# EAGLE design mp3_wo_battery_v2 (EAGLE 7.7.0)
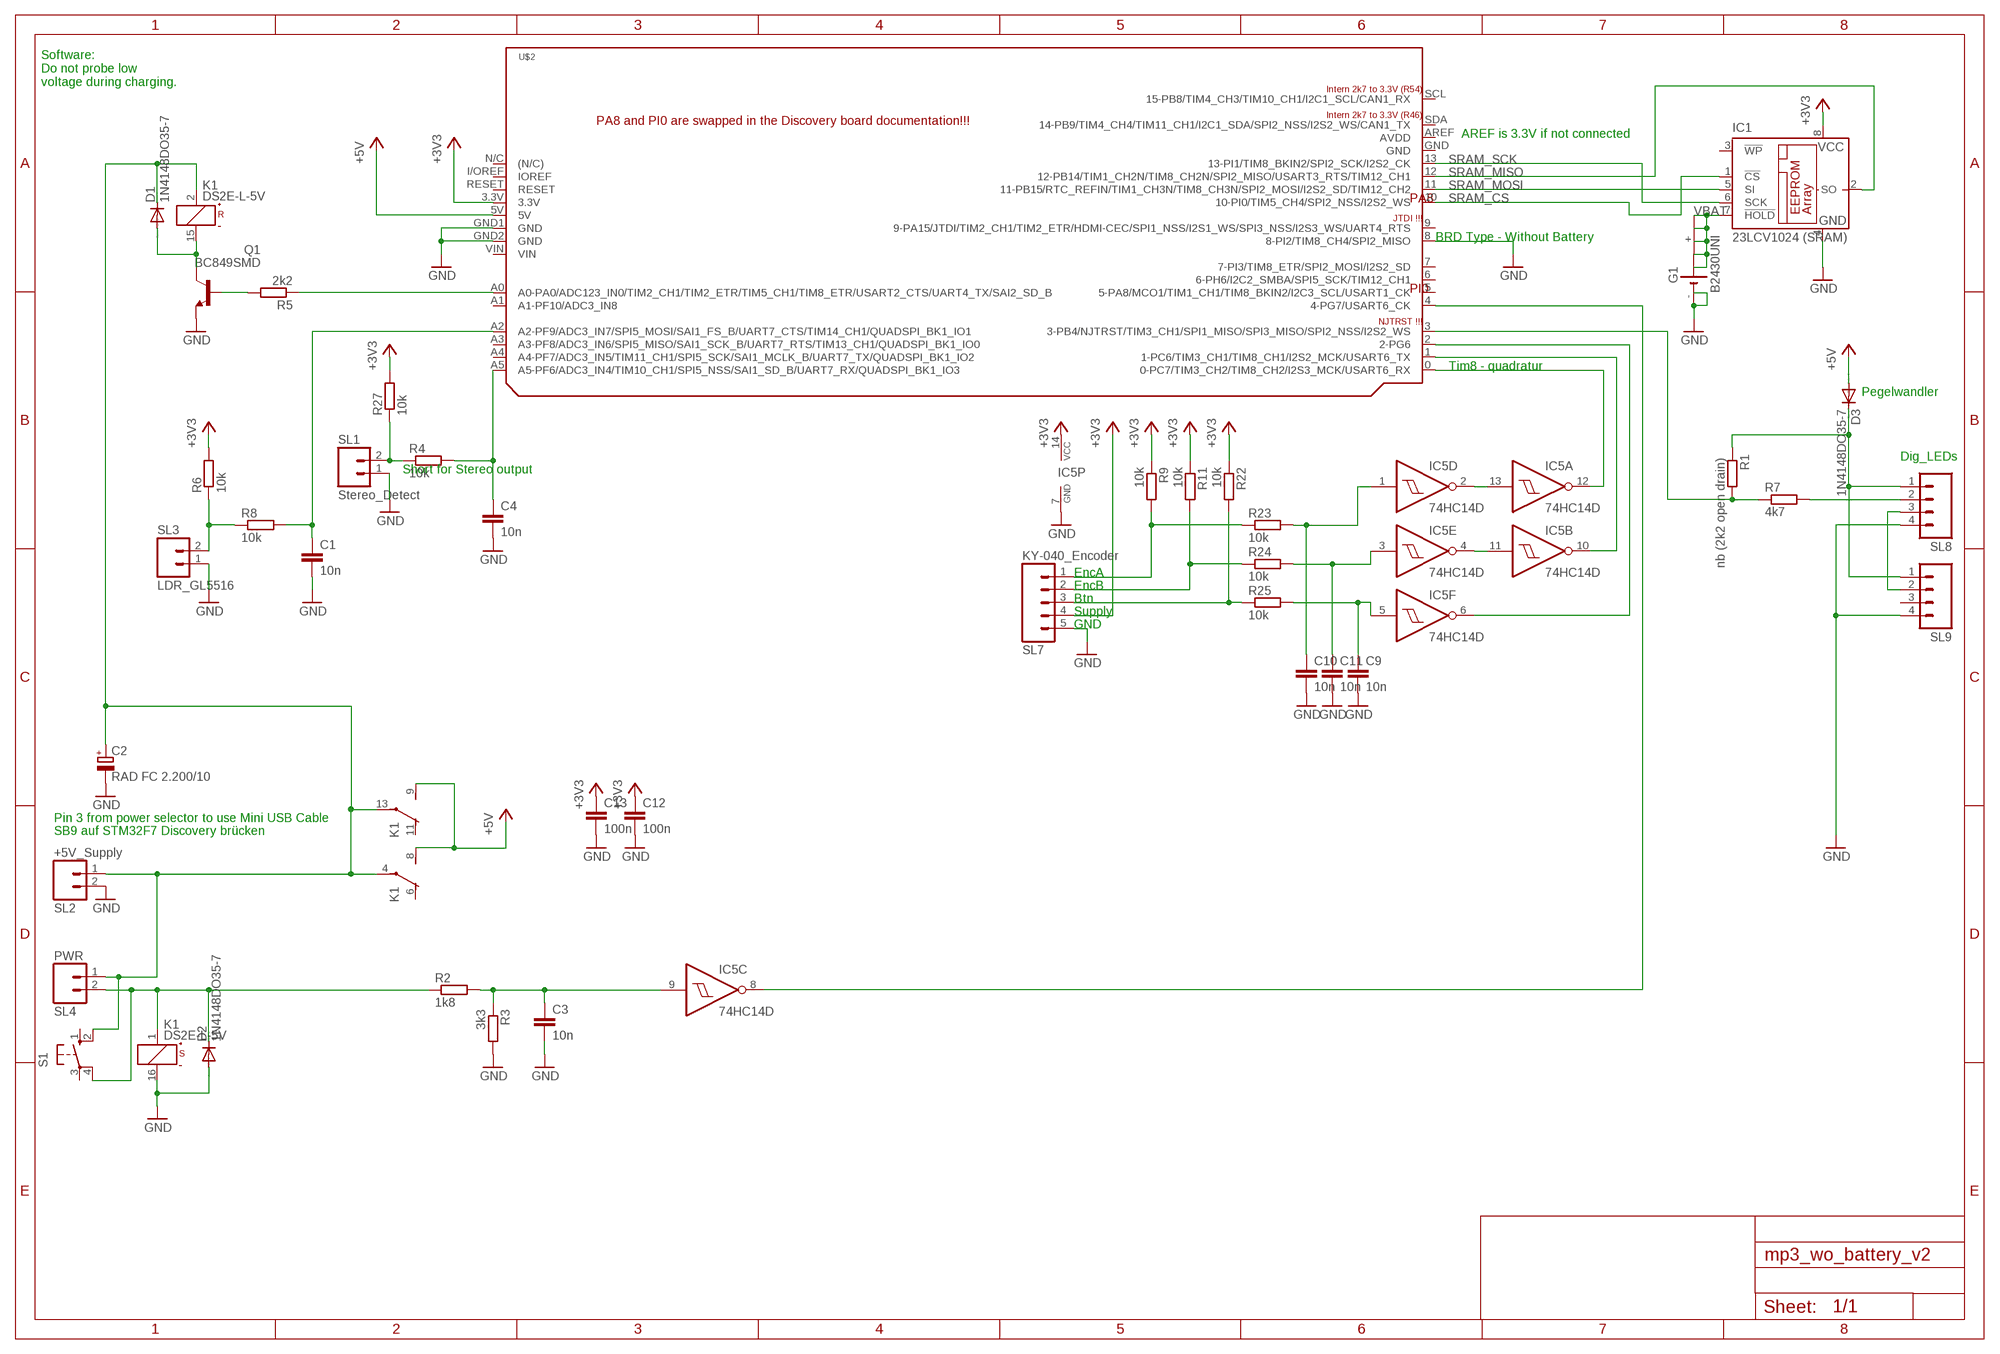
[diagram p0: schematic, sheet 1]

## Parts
C1  10n  C-EUC0805  [C0805]
C2  RAD FC 2.200/10  CPOL-EUE5-10.5  [E5-10,5]
C3  10n  C-EUC0805  [C0805]
C4  10n  C-EUC0805  [C0805]
C9  10n  C-EUC0805  [C0805]
C10  10n  C-EUC0805  [C0805]
C11  10n  C-EUC0805  [C0805]
C12  100n  C-EUC0805  [C0805]
C13  100n  C-EUC0805  [C0805]
D1  1N4148DO35-7  [DO35-7]
D2  1N4148DO35-7  [DO35-7]
D3  1N4148DO35-7  [DO35-7]
G1  B2430UNI  [B2430UNI]
IC1  23LCV1024 (SRAM)  25AA080SN  [SO-08]
IC5  74HC14D  [SO14]
K1  DS2E-L-5V  [DS2E-L]
Q1  BC849SMD  [SOT23-BEC]
R1  nb (2k2 open drain)  R-EU_M0805  [M0805]
R2  1k8  R-EU_M0805  [M0805]
R3  3k3  R-EU_M0805  [M0805]
R4  10k  R-EU_M0805  [M0805]
R5  2k2  R-EU_M0805  [M0805]
R6  10k  R-EU_M0805  [M0805]
R7  4k7  R-EU_M0805  [M0805]
R8  10k  R-EU_M0805  [M0805]
R9  10k  R-EU_M0805  [M0805]
R11  10k  R-EU_M0805  [M0805]
R22  10k  R-EU_M0805  [M0805]
R23  10k  R-EU_M0805  [M0805]
R24  10k  R-EU_M0805  [M0805]
R25  10k  R-EU_M0805  [M0805]
R27  10k  R-EU_M0805  [M0805]
S1  10-XX  [B3F-10XX]
SL1  Stereo_Detect  M02  [02P]
SL2  +5V_Supply  M02  [02P]
SL3  LDR_GL5516  M02  [02P]
SL4  PWR  M02  [02P]
SL7  KY-040_Encoder  M05  [05P]
SL8  M04  [04P]
SL9  M04  [04P]
U$2  STM32F7_DISCO  [STM32F7_DISCO]

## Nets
+3V3: C12.1 C13.1 IC1.8(VCC) IC5.14(P:VCC) R6.2 R9.1 R11.1 R22.1 R27.2 SL7.4 U$2.3.3V
+5V: D3.A K1.8(3:S) K1.9(4:S) U$2.5V
GND: C1.2 C2.- C3.2 C4.2 C9.2 C10.2 C11.2 C12.2 C13.2 D2.A G1.- G1.-@1(-) IC1.4(GND) IC5.7(P:GND) K1.16(2:-) Q1.E R3.2 SL1.1 SL2.2 SL3.1 SL7.5 SL8.4 SL9.4 U$2.8(8-PI2/TIM8_CH4/SPI2_MISO) U$2.GND1(GND) U$2.GND2(GND)
N$1: C3.1 IC5.9(C:I) R2.2 R3.1
N$2: C2.+ D1.C K1.2(1:+) K1.4(3:P) K1.13(4:P) S1.2(S1) SL2.1 SL4.1
N$3: C4.1 R4.2 U$2.A5(A5-PF6/ADC3_IN4/TIM10_CH1/SPI5_NSS/SAI1_SD_B/UART7_RX/QUADSPI_BK1_IO3)
N$4: IC5.8(C:O) U$2.4(4-PG7/USART6_CK)
N$5: IC5.10(B:O) U$2.1(1-PC6/TIM3_CH1/TIM8_CH1/I2S2_MCK/USART6_TX)
N$6: IC5.12(A:O) U$2.0(0-PC7/TIM3_CH2/TIM8_CH2/I2S3_MCK/USART6_RX)
N$7: IC5.6(F:O) U$2.2(2-PG6)
N$8: SL8.3 SL9.2
N$10: R1.2 R7.1 U$2.3(3-PB4/NJTRST/TIM3_CH1/SPI1_MISO/SPI3_MISO/SPI2_NSS/I2S2_WS)
N$12: R5.1 U$2.A0(A0-PA0/ADC123_IN0/TIM2_CH1/TIM2_ETR/TIM5_CH1/TIM8_ETR/USART2_CTS/UART4_TX/SAI2_SD_B)
N$13: Q1.B R5.2
N$14: D1.A K1.15(1:-) Q1.C
N$15: C1.1 R8.2 U$2.A2(A2-PF9/ADC3_IN7/SPI5_MOSI/SAI1_FS_B/UART7_CTS/TIM14_CH1/QUADSPI_BK1_IO1)
N$16: D3.C R1.1 SL8.1 SL9.1
N$17: R7.2 SL8.2
N$18: R6.1 R8.1 SL3.2
N$26: R9.2 R23.1 SL7.1
N$28: R11.2 R24.1 SL7.2
N$30: R22.2 R25.1 SL7.3
N$31: IC5.2(D:O) IC5.13(A:I)
N$32: IC5.4(E:O) IC5.11(B:I)
N$34: C9.1 IC5.5(F:I) R25.2
N$35: R4.1 R27.1 SL1.2
N$36: C11.1 IC5.3(E:I) R24.2
N$37: C10.1 IC5.1(D:I) R23.2
PWRBTN: D2.C K1.1(2:+) R2.1 S1.4(P1) SL4.2
SRAM_CS: IC1.1(!CS) U$2.10(10-PI0/TIM5_CH4/SPI2_NSS/I2S2_WS)
SRAM_MISO: IC1.2(SO) U$2.12(12-PB14/TIM1_CH2N/TIM8_CH2N/SPI2_MISO/USART3_RTS/TIM12_CH1)
SRAM_MOSI: IC1.5(SI) U$2.11(11-PB15/RTC_REFIN/TIM1_CH3N/TIM8_CH3N/SPI2_MOSI/I2S2_SD/TIM12_CH2)
SRAM_SCK: IC1.6(SCK) U$2.13(13-PI1/TIM8_BKIN2/SPI2_SCK/I2S2_CK)
VBAT: G1.+ G1.+@1(+) G1.+@2(+) G1.+@3(+) G1.+@4(+) IC1.7(!HOLD)
Unconnected: IC1.3(!WP) K1.6(3:O) K1.11(4:O) S1.1(S) S1.3(P) SL9.3 U$2.5(5-PA8/MCO1/TIM1_CH1/TIM8_BKIN2/I2C3_SCL/USART1_CK) U$2.6(6-PH6/I2C2_SMBA/SPI5_SCK/TIM12_CH1) U$2.7(7-PI3/TIM8_ETR/SPI2_MOSI/I2S2_SD) U$2.9(9-PA15/JTDI/TIM2_CH1/TIM2_ETR/HDMI-CEC/SPI1_NSS/I2S1_WS/SPI3_NSS/I2S3_WS/UART4_RTS) U$2.A1(A1-PF10/ADC3_IN8) U$2.A3(A3-PF8/ADC3_IN6/SPI5_MISO/SAI1_SCK_B/UART7_RTS/TIM13_CH1/QUADSPI_BK1_IO0) U$2.A4(A4-PF7/ADC3_IN5/TIM11_CH1/SPI5_SCK/SAI1_MCLK_B/UART7_TX/QUADSPI_BK1_IO2) U$2.AREF(AVDD) U$2.GND U$2.I/OREF(IOREF) U$2.N/C((N/C)) U$2.RESET U$2.SCL(15-PB8/TIM4_CH3/TIM10_CH1/I2C1_SCL/CAN1_RX) U$2.SDA(14-PB9/TIM4_CH4/TIM11_CH1/I2C1_SDA/SPI2_NSS/I2S2_WS/CAN1_TX) U$2.VIN

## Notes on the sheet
- Software:
  Do not probe low 
  voltage during charging.
- AREF is 3.3V if not connected
- BRD Type - Without Battery
- Tim8 - quadratur
- Pegelwandler
- Dig_LEDs
- Short for Stereo output
- EncA
- EncB
- Btn
- Supply
- GND
- Pin 3 from power selector to use Mini USB Cable
- SB9 auf STM32F7 Discovery brücken

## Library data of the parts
C1 C3 C4 C9-C13 = rcl:C-EU: CAPACITOR, European symbol
C2 = rcl:CPOL-EU: POLARIZED CAPACITOR, European symbol
D1-D3 = diode:1N4148: DIODE
G1 = battery:B2430UNI: LI BATTERY
IC1 = microchip:25*: Serial EEPROM 4K/ 8K , SPI bus; MF: MICROCHIP; MPN: 25AA080/SN; OC_FARNELL: 1816072; OC_NEWARK: 92C7351
IC5 = 74xx-eu:74*14: Hex schmitt trigger INVERTER
K1 = relay:DS2E-L-*: DS-RELAYS HIGHLY SENSITIVE 1500 V FCC SURGE NAiS WITHSTANDING MINIATURE RELAY Source: Panasonic data sheet; MF: AROMAT/ MATSUSHITA; MPN: DS2E-SL-DC5V; OC_FARNELL: unknown; OC_NEWARK: 10C5815
Q1 = transistor-npn:BC849*: NPN Transistor
R1-R9 R11 R22-R25 R27 = rcl:R-EU_: RESISTOR, European symbol
S1 = switch-omron:10-XX: OMRON SWITCH; MPN: B3F-1000; OC_FARNELL: 176432; OC_NEWARK: 36M3542
SL1-SL4 = con-amp-quick:M02: AMP QUICK CONNECTOR; OC_FARNELL: unknown; OC_NEWARK: unknown
SL7 = con-amp-quick:M05: AMP QUICK CONNECTOR; OC_FARNELL: unknown; OC_NEWARK: unknown
SL8 SL9 = con-amp-quick:M04: AMP QUICK CONNECTOR; OC_FARNELL: unknown; OC_NEWARK: unknown
U$2 = stm32f7_disco:STM32F7_DISCO

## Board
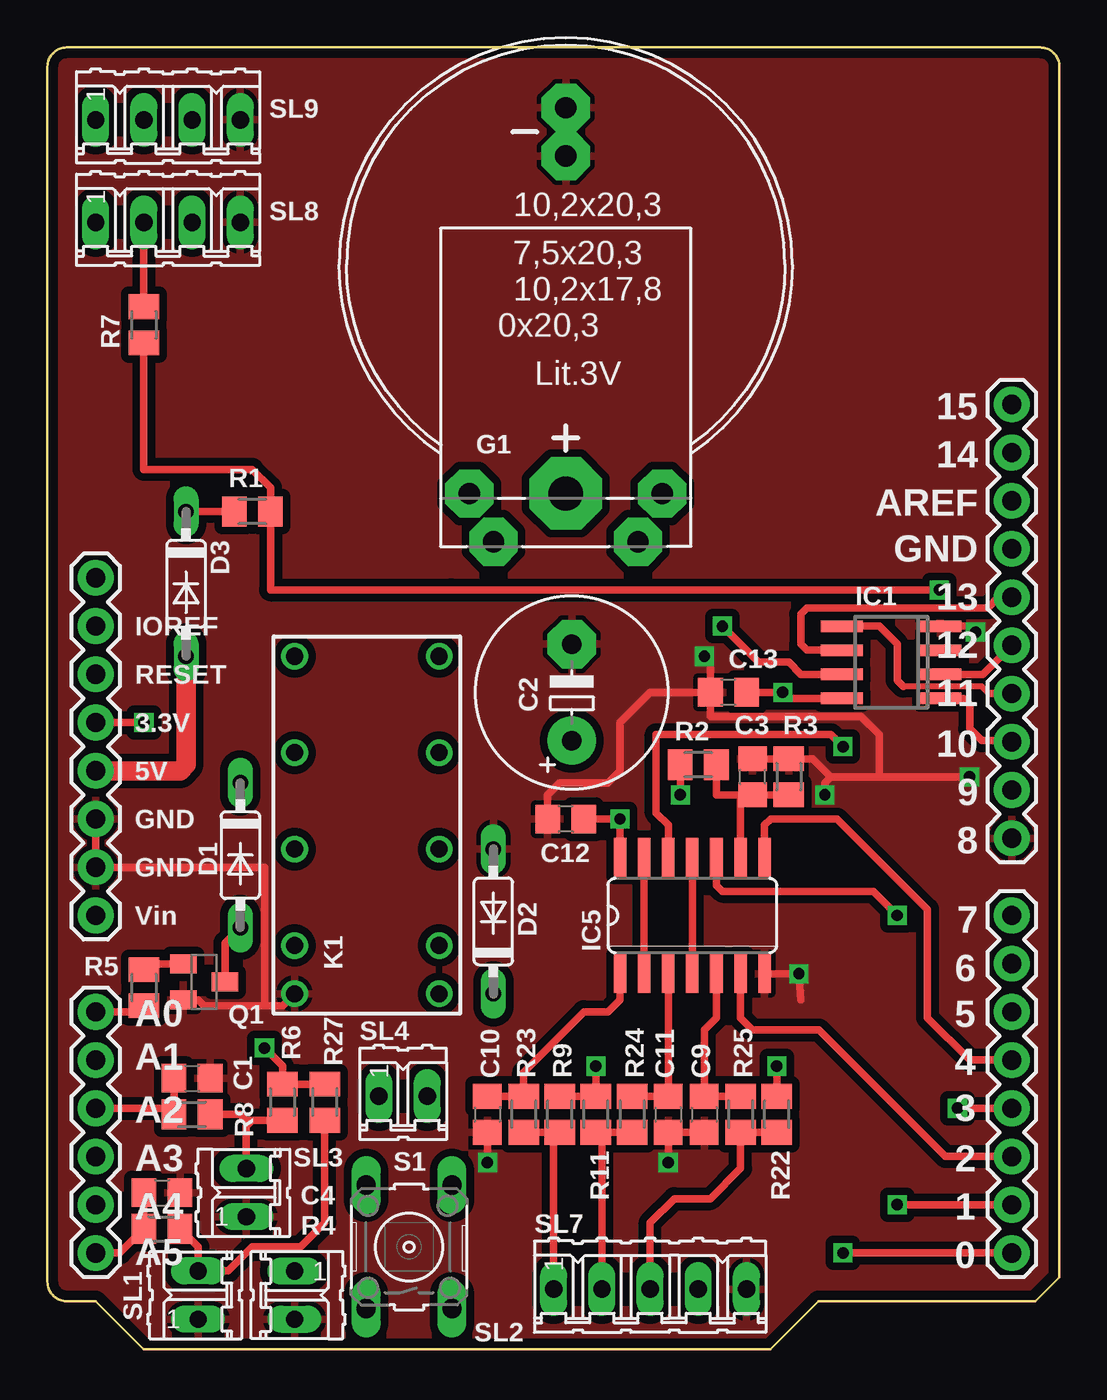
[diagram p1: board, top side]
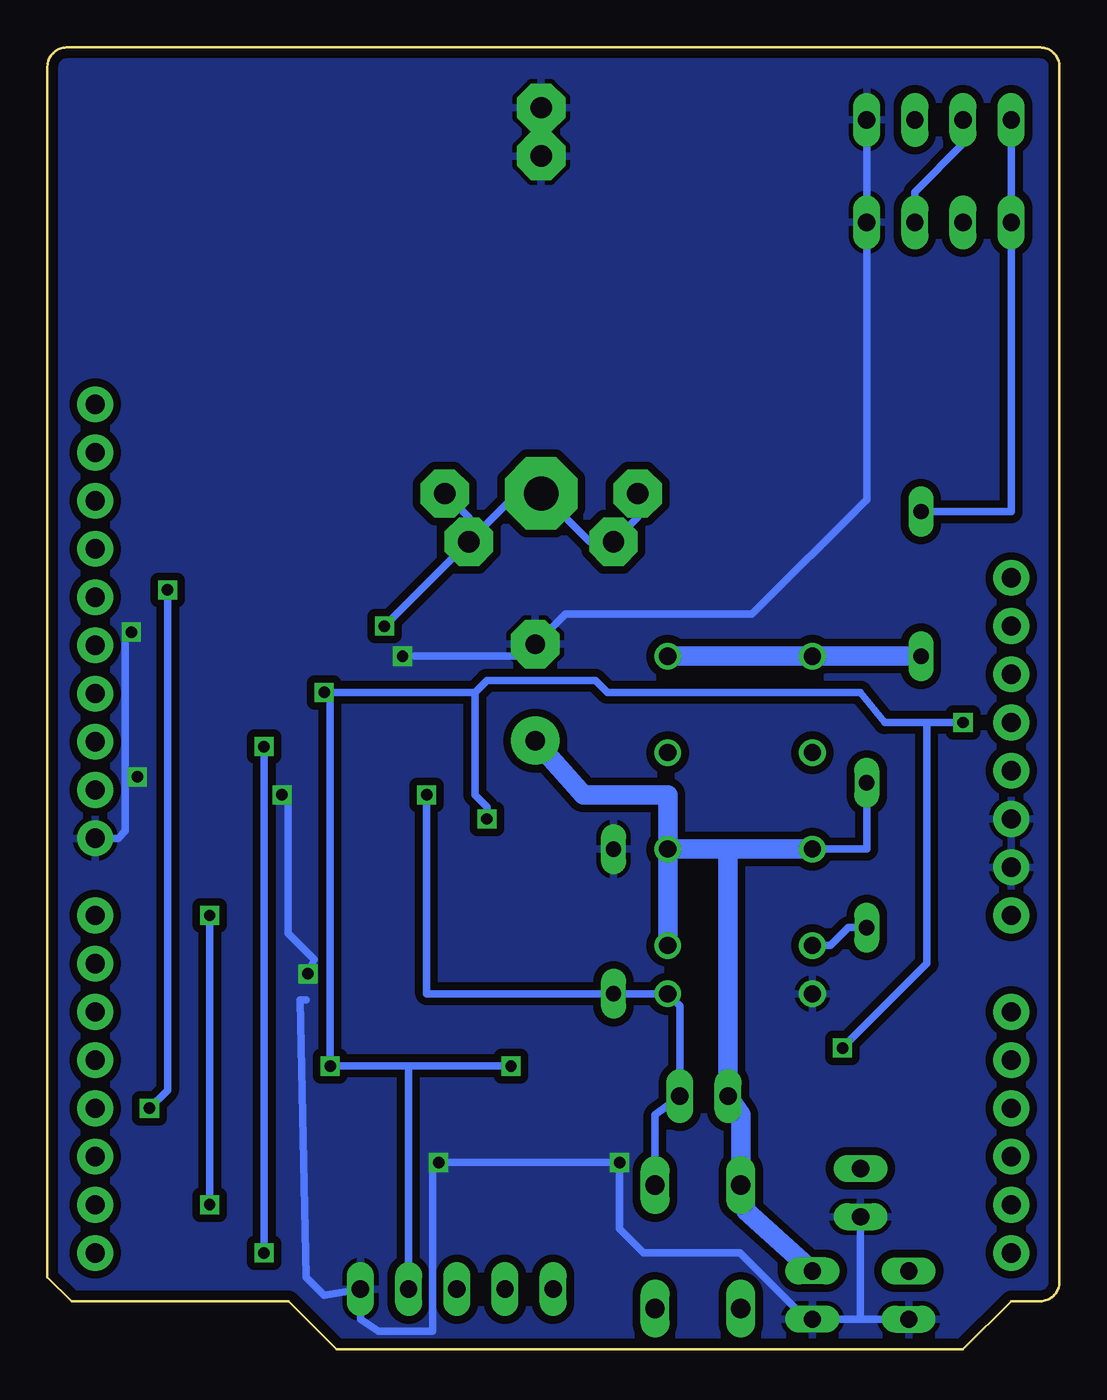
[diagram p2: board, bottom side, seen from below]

Size 53.31 x 68.58 mm. Coordinates in mm from the lower left corner, seen from the top.
Copper layers (1*16): Top 0.035mm / dielectric 1.5mm / Bottom 0.035mm
Design rules "default *": minimum track width 0.2mm, minimum drill 0.6mm, track to track 8mil, track to pad 8mil, pad to pad 8mil, via to via 8mil, smd to smd 8mil, copper to edge 0.5mm, drill to drill 8mil, minimum pad ring 10mil, minimum via ring 8mil, stop-mask expansion 4mil, vias tented up to drill 0mil, thermal gap 10mil

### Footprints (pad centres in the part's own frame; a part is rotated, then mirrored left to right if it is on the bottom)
C0805 = smd 1.3 x 1.5: 1 -0.95,0; 2 0.95,0
E5-10,5 = drill 1.016 pad 2.54: + -2.54,0 | drill 1.016 pad 2.54 octagon: - 2.54,0
DO35-7 = drill 0.813 long: A 3.81,0; C -3.81,0
B2430UNI = drill 1.118 pad 2.54 octagon: + 3.81,14.605; +@1 -3.81,14.605; +@2 -5.08,12.065; +@3 5.08,12.065; - 0,-5.715; -@1 0,-8.255 | drill 1.803 pad 3.81 octagon: +@4 0,12.065
SO-08 = smd 0.6 x 2.2: 1 -1.905,-2.6; 2 -0.635,-2.6; 3 0.635,-2.6; 4 1.905,-2.6; 5 1.905,2.6; 6 0.635,2.6; 7 -0.635,2.6; 8 -1.905,2.6
SO14 = smd 0.66 x 2.032: 1 -3.81,-3.073; 2 -2.54,-3.073; 3 -1.27,-3.073; 4 0,-3.073; 5 1.27,-3.073; 6 2.54,-3.073; 7 3.81,-3.073; 8 3.81,3.073; 9 2.54,3.073; 10 1.27,3.073; 11 0,3.073; 12 -1.27,3.073; 13 -2.54,3.073; 14 -3.81,3.073
DS2E-L = drill 0.9: 1 -8.89,-3.81; 2 -6.35,-3.81; 4 -1.27,-3.81; 6 3.81,-3.81; 8 8.89,-3.81; 9 8.89,3.81; 11 3.81,3.81; 13 -1.27,3.81; 15 -6.35,3.81; 16 -8.89,3.81
SOT23-BEC = smd 1 x 1.4: B -0.95,-1.1; C 0,1.1; E 0.95,-1.1
M0805 = smd 1.3 x 1.6: 1 -0.95,0; 2 0.95,0
B3F-10XX = drill 1.016 long: 1 -3.251,2.261; 2 3.251,2.261; 3 -3.251,-2.261; 4 3.251,-2.261
02P = drill 0.914 long: 1 -1.27,0; 2 1.27,0
05P = drill 0.914 long: 1 -5.08,0; 2 -2.54,0; 3 0,0; 4 2.54,0; 5 5.08,0
04P = drill 0.914 long: 1 -3.81,0; 2 -1.27,0; 3 1.27,0; 4 3.81,0
STM32F7_DISCO = drill 1.016 pad 1.88: 0 22.86,-24.13; 1 22.86,-21.59; 2 22.86,-19.05; 3 22.86,-16.51; 3.3V -25.4,3.81; 4 22.86,-13.97; 5 22.86,-11.43; 5V -25.4,1.27; 6 22.86,-8.89; 7 22.86,-6.35; 8 22.86,-2.286; 9 22.86,0.254; 10 22.86,2.794; 11 22.86,5.334; 12 22.86,7.874; 13 22.86,10.414; A0 -25.4,-11.43; A1 -25.4,-13.97; A2 -25.4,-16.51; A3 -25.4,-19.05; A4 -25.4,-21.59; A5 -25.4,-24.13; AREF 22.86,15.494; GND 22.86,12.954; GND1 -25.4,-3.81; GND2 -25.4,-1.27; I/OREF -25.4,8.89; N/C -25.4,11.43; RESET -25.4,6.35; SCL 22.86,20.574; SDA 22.86,18.034; VIN -25.4,-6.35

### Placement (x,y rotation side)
C1  7.62,14.29 0 top
C2  27.62,34.61 90 top
C3  37.15,30.16 90 top
C4  6.03,8.26 0 top
C9  34.61,12.38 270 top
C10  23.18,12.38 270 top
C11  32.7,12.38 270 top
C12  27.3,27.94 180 top
C13  35.88,34.61 180 top
D1  10.16,26.04 270 top
D2  23.5,22.54 90 top
D3  7.3,40.32 270 top
G1  27.3,57.15 180 top
IC1  44.45,36.2 90 top
IC5  33.97,22.86 0 top
K1  16.83,27.62 90 top
Q1  8.26,19.37 270 top
R1  10.79,44.13 0 top
R2  34.29,30.8 0 top
R3  39.05,30.16 90 top
R4  6.03,6.35 180 top
R5  5.08,19.05 90 top
R6  12.38,13.02 90 top
R7  5.08,53.98 90 top
R8  7.62,12.38 180 top
R9  26.99,12.38 270 top
R11  28.89,12.38 270 top
R22  38.42,12.38 270 top
R23  25.08,12.38 90 top
R24  30.8,12.38 90 top
R25  36.51,12.38 90 top
R27  14.61,13.02 90 top
S1  19.05,5.4 90 top
SL1  7.94,2.86 90 top
SL2  13.02,2.86 270 top
SL3  10.48,8.26 90 top
SL4  18.73,13.34 0 top
SL7  31.75,3.17 0 top
SL8  6.35,59.37 0 top
SL9  6.35,64.77 0 top
U$2  27.94,29.21 0 top

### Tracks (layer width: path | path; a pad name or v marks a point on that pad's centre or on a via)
+3V3  (via drill 0.6)
  Top 0.406: U$2.3.3V v5.08,33.02 | IC1.8 39.05,34.29 v38.73,34.61 C13.1 | R9.1 R11.1 v28.89,14.92 | v38.42,14.92 R22.1 | IC5.14 v30.16,27.94 C12.1 | R27.2 R6.2 12.38,14.92 v11.43,15.88
  Bottom 0.406: v5.08,33.02 6.99,33.02 | 6.99,33.02 9.21,33.02 10.48,34.61 23.81,34.61 24.45,35.24 30.16,35.24 30.8,34.61 | 30.8,34.61 38.42,34.61 | v11.43,15.88 6.99,20.32 6.99,33.02 | v38.73,34.61 38.42,34.61 | v28.89,14.92 34.29,14.92 | 34.29,14.92 v38.42,14.92 38.42,34.61 | SL7.4 34.29,14.92 | v30.16,27.94 30.16,28.57 30.8,29.21 30.8,34.61
+5V
  Top 1.016: U$2.5V 6.99,30.48 7.3,30.8 D3.A
  Bottom 1.016: K1.8 K1.9 D3.A
GND  (via drill 0.6)
  Top 0.406: IC5.7 v39.59,19.79 39.69,18.41 | IC1.4 48.58,38.1 v48.9,37.78 | U$2.GND2 U$2.GND1 11.43,25.4 11.43,18.1 | C13.2 34.93,36.19 v34.61,36.51 | C13.2 31.75,34.61 30.16,33.02 30.16,30.48 29.53,29.84 26.99,29.84 26.35,29.21 C12.2 | C3.2 R3.2 40.33,31.11 41.27,30.16 | 41.27,30.16 43.81,30.16 | 43.81,30.16 v48.58,30.16 | v40.96,29.21 40.96,29.84 41.27,30.16 | C13.2 34.93,33.34 34.92,33.34 42.86,33.34 43.81,32.38 43.81,30.16 | C10.2 v23.18,9.84 | v32.7,9.84 C11.2 C9.2 | Q1.E 7.93,18.42 8.26,18.1 11.43,18.1 | 11.43,18.1 12.38,18.1 K1.16
  Bottom 0.406: 39.69,18.41 40.01,18.41 39.69,3.81 38.73,2.86 SL7.5 36.83,1.59 35.88,0.95 33.02,0.95 33.02,9.53 v32.7,9.84 v23.18,9.84 23.18,6.35 21.91,5.08 16.83,5.08 13.34,1.59 SL2.2 10.48,1.59 | SL9.4 SL8.4 10.16,44.77 16.19,38.73 26.04,38.73 C2.- 28.26,36.51 v34.61,36.51 | U$2.8 49.59,26.92 49.21,27.3 49.21,30.16 | 49.21,30.16 49.21,37.47 v48.9,37.78 | v48.58,30.16 49.21,30.16 | v39.59,19.79 39.27,20.54 40.64,21.91 40.64,28.89 v40.96,29.21 | G1.-@1 G1.- | SL1.1 10.48,1.59 | SL3.1 10.48,1.59
  pour Bottom (isolate 0.406): -3.49,72.71 58.74,72.71 58.74,-1.27 -3.49,-1.27
  pour Top (isolate 0.406): -0.64,0 54.93,0 54.61,70.17 -0.64,70.17
N$1
  Top 0.406: IC5.9 36.51,29.21 C3.1 | C3.1 R3.1 | R2.2 35.24,29.21 C3.1
N$2
  Bottom 0.406: K1.13 10.16,26.35 D1.C
  Bottom 1.016: K1.13 17.46,26.35 | 17.46,26.35 K1.4 | K1.4 K1.2 | K1.4 20.64,29.21 25.08,29.21 C2.+ | 17.46,26.35 SL4.1 16.79,12.34 S1.2 16.59,8.65 16.51,7.3 SL2.1
N$3
  Top 0.406: U$2.A5 3.81,5.08 R4.2 C4.1
N$4
  Top 0.406: IC5.8 37.78,27.62 38.1,27.94 41.59,27.94 46.35,23.18 46.35,17.46 48.58,15.24 U$2.4
N$5  (via drill 0.6)
  Top 0.406: IC5.10 35.24,24.45 35.56,24.13 43.5,24.13 v44.77,22.86 | v44.77,7.62 U$2.1
  Bottom 0.406: v44.77,22.86 v44.77,7.62
N$6  (via drill 0.6)
  Top 0.406: IC5.12 32.7,27.62 32.07,28.26 32.07,32.38 41.27,32.38 v41.91,31.75 | v41.91,5.08 U$2.0
  Bottom 0.406: v41.91,31.75 v41.91,5.08
N$7
  Top 0.406: IC5.6 36.51,17.46 37.15,16.83 40.64,16.83 47.31,10.16 U$2.2
N$8
  Bottom 0.406: SL9.2 5.08,63.5 7.62,60.96 SL8.3
N$10  (via drill 0.6)
  Top 0.406: v46.99,40.01 21.27,40.01 11.75,40 R1.2 11.74,45.41 10.79,46.35 5.08,46.35 R7.1 | v47.94,12.7 U$2.3
  Bottom 0.406: v46.99,40.01 46.99,13.65 v47.94,12.7
N$12
  Top 0.406: U$2.A0 5.08,17.78 R5.1
N$13
  Top 0.406: R5.2 5.4,20.32 Q1.B
N$14
  Top 0.406: Q1.C 9.36,21.42 D1.A
  Bottom 0.406: K1.15 12.06,21.27 11.11,22.23 D1.A
N$15
  Top 0.406: U$2.A2 6.35,12.7 R8.2 C1.1
N$16
  Top 0.406: R1.1 D3.C
  Bottom 0.406: SL9.1 SL8.1 2.54,44.13 D3.C
N$17
  Top 0.406: SL8.2 R7.2
N$18
  Top 0.406: R8.1 10.16,12.38 10.48,12.06 10.79,12.06 | 10.79,12.06 R6.1 | SL3.2 10.48,11.75 10.79,12.06
N$26
  Top 0.406: R23.1 R9.2 26.67,11.12 SL7.1
N$28
  Top 0.406: SL7.2 29.21,11.12 R11.2 R24.1
N$30
  Top 0.406: SL7.3 31.75,6.67 33.02,7.94 34.92,7.94 36.51,9.53 R25.1 R22.2
N$31
  Top 0.406: IC5.2 IC5.13
N$32
  Top 0.406: IC5.4 IC5.11
N$34
  Top 0.406: R25.2 C9.1 34.61,16.83 35.24,17.46 IC5.5
N$35
  Top 0.406: R4.1 7.94,5.39 SL1.2 9.53,4.13 10.79,5.4 13.34,5.4 14.61,6.67 R27.1
N$36
  Top 0.406: R24.2 C11.1 IC5.3
N$37
  Top 0.406: C10.1 R23.2 25.08,14.61 28.26,17.78 29.53,17.78 30.16,18.41 IC5.1
PWRBTN  (via drill 0.6)
  Top 0.406: v33.34,29.21 33.34,30.48 R2.1
  Bottom 0.406: S1.4 21.31,12.34 SL4.2 20,18.1 K1.1 D2.C 33.34,18.73 v33.34,29.21
SRAM_CS
  Top 0.406: IC1.1 48.26,34.29 48.58,33.97 48.58,32.7 49.21,32.07 50.74,32.07 U$2.10
SRAM_MISO
  Top 0.406: IC1.2 49.28,35.56 U$2.12
SRAM_MOSI
  Top 0.305: 49.59,34.54 49.21,34.92 45.09,34.92
  Top 0.406: U$2.11 49.59,34.54 | 45.09,34.92 44.77,35.24 44.77,37.15 43.81,38.1 42.23,38.1 IC1.5
SRAM_SCK
  Top 0.406: U$2.13 50.1,39.62 49.53,39.05 40.01,39.05 39.69,38.73 39.69,37.15 40.01,36.83 IC1.6
VBAT  (via drill 0.6)
  Top 0.406: v35.56,38.1 37.47,36.2 39.05,36.2 39.69,35.56 IC1.7
  Bottom 0.406: G1.+@3 22.23,43.81 G1.+ 24.77,42.55 G1.+@4 28.57,45.09 G1.+@1 | G1.+@1 31.11,43.81 G1.+@2 | G1.+@1 v35.56,38.1

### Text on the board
tDocu: MP3-Player V2 / Daniel Schramm / pinguin.sauerland.de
